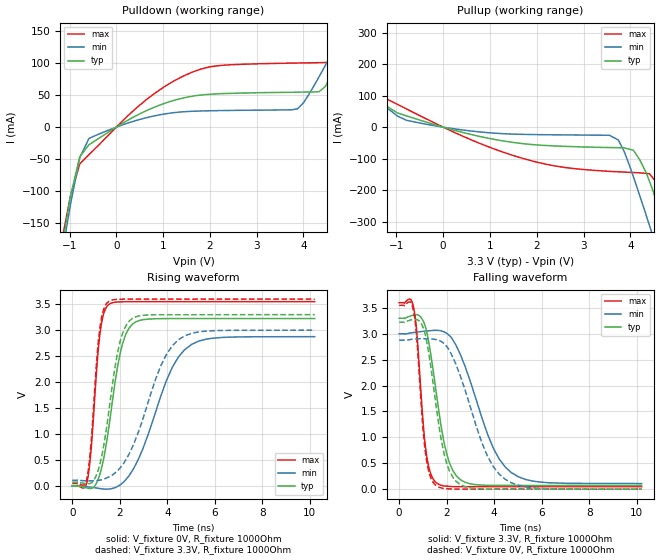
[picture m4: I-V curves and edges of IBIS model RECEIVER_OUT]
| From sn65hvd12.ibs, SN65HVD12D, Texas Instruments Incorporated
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|   Receiver Output Model
[Model]   RECEIVER_OUT
Model_type   Output
| Signals   R
Vmeas = 1.65V   |Reference voltage for timing measurements
Cref = 15pF   |Timing specification test load capacitance value
Vref = 0V   |Timing specification test load voltage; GND
| variable   typ   min   max
|C_Comp output low
C_comp   11.07pF   11.88pF   9.90pF
|C_comp output high
|C_comp   13.14pF   13.54pF   11.73pF
|   typ   min   max
[Temperature Range]   25.0   85   -40
[Voltage range]   3.3V   3.0V   3.6V
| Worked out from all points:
|   slope of the pulldown table from 0 to 0.495 V, typ, clamps not added: 24.1 ohm
|   slope of the pullup table from 0 to 0.495 V, typ, clamps not added: 25.1 ohm
|   falling waveform, V_fixture 3.3V, R_fixture 1000Ohm: 20-80 % time 672ps typ, 1.36ns min, 358ps max; typ from 3.3 V to 0.071 V
|   rising waveform, V_fixture 0V, R_fixture 1000Ohm: 20-80 % time 658ps typ, 1.39ns min, 349ps max; typ from 0 V to 3.22 V
|   rising waveform, V_fixture 3.3V, R_fixture 1000Ohm: 20-80 % time 650ps typ, 1.38ns min, 345ps max; typ from 0.071 V to 3.3 V
|   falling waveform, V_fixture 0V, R_fixture 1000Ohm: 20-80 % time 652ps typ, 1.31ns min, 349ps max; typ from 3.22 V to 0 V
[Pulldown]
|   Voltage   I(typ)   I(min)   I(max)
-3.3V     -1.262A    -1.197A    -1.336A
-1.178V   -195.4mA   -206.9mA   -182.4mA
-979.8mV  -107.7mA   -120.7mA   -107.6mA
-781.8mV  -46.3mA    -47.69mA   -57.5mA
-583.8mV  -27.47mA   -17.6mA    -42.96mA
634.9mV   25.36mA    14.58mA    42.44mA
1.625V    48.21mA    24.76mA    85.92mA
3.873V    54.57mA    28.56mA    100.1mA
4.467V    63.49mA    96.34mA    100.8mA
4.908V    133.4mA    156.3mA    106.3mA
5.284V    199mA      208.2mA    170.2mA
6.6V      434.2mA    392.3mA    469.4mA
[Pullup]
|   Voltage   I(typ)   I(min)   I(max)
-3.3V     434.2mA    350.2mA    538.7mA
-2.762V   337.5mA    274.8mA    414.7mA
-2.366V   266.8mA    219.7mA    323.8mA
-1.376V   94.17mA    84.21mA    108.1mA
-781.8mV  35.66mA    21.58mA    57.58mA
1.625V    -51mA      -22.69mA   -95.98mA
3.742V    -65.45mA   -40.5mA    -141.8mA
4.067V    -73.52mA   -158.2mA   -144.1mA
4.467V    -194.5mA   -339mA     -159mA
4.754V    -331.5mA   -472.6mA   -238.4mA
4.988V    -448.2mA   -582.1mA   -315.9mA
6.6V      -1.262A    -1.338A    -1.171A
[Ramp]
R_load = 1000
|   typ   min   max
dV/dt_r   1.93447/6.58356e-010   1.72549/1.3901e-009   2.1301/3.48637e-010
dV/dt_f   1.93753/6.71847e-010   1.73539/1.35739e-009   2.13143/3.58068e-010
[Falling Waveform]
V_fixture = 3.3V
V_fixture_min = 3V
V_fixture_max = 3.6V
R_fixture = 1000Ohm
C_fixture = 0F
|   Time   V(typ)   V(min)   V(max)
0s        3.3V       3V         3.6V
609.2ps   3.361V     3.025V     3.508V
721.4ps   3.369V     3.031V     3.139V
1.163ns   3.027V     3.054V     625.3mV
1.624ns   1.659V     3.065V     102.9mV
2.006ns   674.2mV    3.007V     57.6mV
2.39ns    267.6mV    2.783V     48.19mV
3.97ns    72.27mV    786.6mV    48.07mV
4.718ns   72.09mV    321.7mV    48.01mV
10.21ns   70.78mV    107.7mV    47.61mV
[Rising Waveform]
V_fixture = 0V
V_fixture_min = 0V
V_fixture_max = 0V
R_fixture = 1000Ohm
C_fixture = 0F
|   Time   V(typ)   V(min)   V(max)
0s        624.3pV    1.026nV    384.1pV
609.2ps   -39.66mV   -16.3mV    51.15mV
797.8ps   -48.02mV   -26.55mV   729mV
1.163ns   225.3mV    -51.3mV    2.926V
1.534ns   1.111V     -60.44mV   3.494V
2.116ns   2.741V     56.75mV    3.547V
2.664ns   3.158V     405.6mV    3.55V
4.219ns   3.224V     2.291V     3.55V
5.023ns   3.224V     2.726V     3.55V
10.21ns   3.224V     2.876V     3.55V
[Rising Waveform]
V_fixture = 3.3V
V_fixture_min = 3V
V_fixture_max = 3.6V
R_fixture = 1000Ohm
C_fixture = 0F
|   Time   V(typ)   V(min)   V(max)
0s        70.78mV    107.5mV    47.61mV
609.2ps   43.99mV    98.4mV     125.3mV
759.6ps   48.58mV    97.35mV    657.9mV
1.163ns   421mV      110.5mV    3.048V
1.534ns   1.421V     171.3mV    3.554V
2.006ns   2.77V      341.4mV    3.596V
2.39ns    3.172V     611.3mV    3.6V
3.721ns   3.298V     2.307V     3.6V
4.468ns   3.298V     2.815V     3.6V
10.21ns   3.3V       3V         3.6V
[Falling Waveform]
|Gnd
V_fixture = 0V
V_fixture_min = 0V
V_fixture_max = 0V
R_fixture = 1000Ohm
C_fixture = 0F
|   Time   V(typ)   V(min)   V(max)
0s        3.224V     2.876V     3.55V
609.2ps   3.276V     2.896V     3.437V
721.4ps   3.277V     2.9V       3.028V
1.104ns   2.973V     2.904V     706mV
1.534ns   1.683V     2.89V      77.74mV
1.896ns   674.1mV    2.811V     12.27mV
2.39ns    155.1mV    2.411V     373.9uV
3.721ns   1.945mV    635.3mV    310.3uV
4.468ns   -413uV     189.5mV    274.6uV
10.21ns   88.8nV     37.29uV    30.2nV
